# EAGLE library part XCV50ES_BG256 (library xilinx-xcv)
xcv50es_bg256 edit this description Auto generated by make-symbol-device-package-bsdl.ulp Rev. 26 Source: xcv50es_bg256.bsd
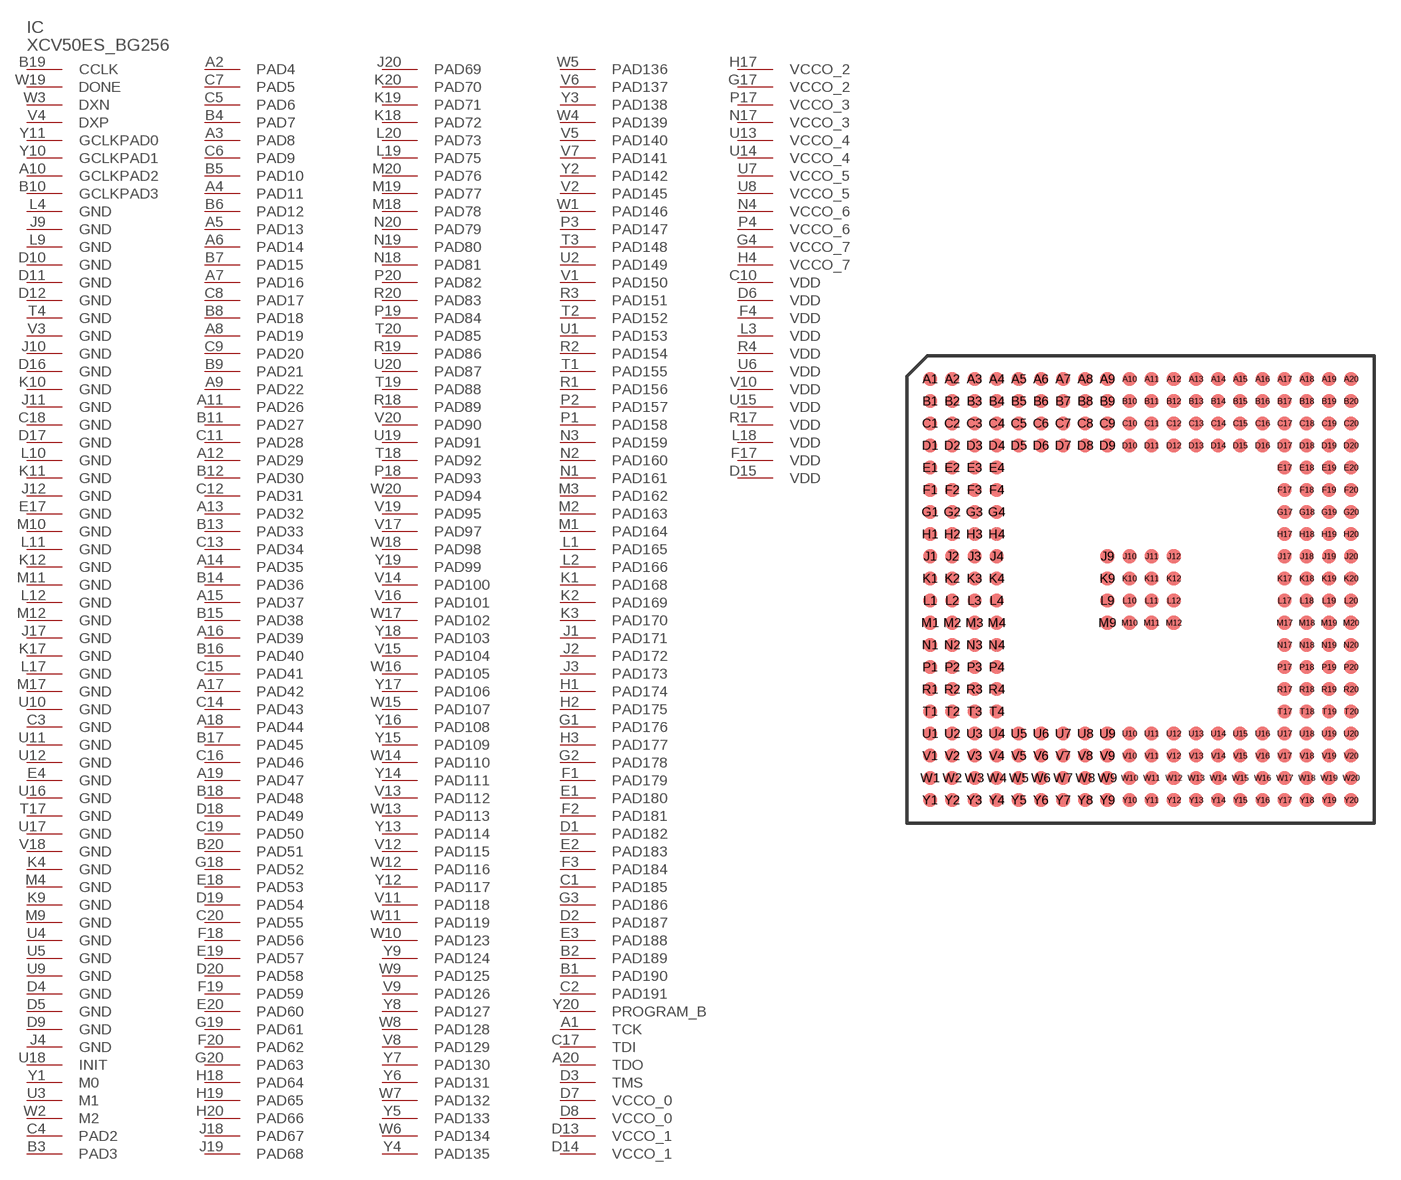
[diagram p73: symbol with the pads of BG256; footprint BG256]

Designator prefix IC

## XCV50ES_BG256 (OC_FARNELL: unknown; OC_NEWARK: unknown)  [BG256]
A1  TCK  in
A2  PAD4
A3  PAD8
A4  PAD11
A5  PAD13
A6  PAD14
A7  PAD16
A8  PAD19
A9  PAD22
A10  GCLKPAD2  in
A11  PAD26
A12  PAD29
A13  PAD32
A14  PAD35
A15  PAD37
A16  PAD39
A17  PAD42
A18  PAD44
A19  PAD47
A20  TDO  out
B1  PAD190
B2  PAD189
B3  PAD3
B4  PAD7
B5  PAD10
B6  PAD12
B7  PAD15
B8  PAD18
B9  PAD21
B10  GCLKPAD3  in
B11  PAD27
B12  PAD30
B13  PAD33
B14  PAD36
B15  PAD38
B16  PAD40
B17  PAD45
B18  PAD48
B19  CCLK
B20  PAD51
C1  PAD185
C2  PAD191
C3  GND  pwr
C4  PAD2
C5  PAD6
C6  PAD9
C7  PAD5
C8  PAD17
C9  PAD20
C10  VDD  pwr
C11  PAD28
C12  PAD31
C13  PAD34
C14  PAD43
C15  PAD41
C16  PAD46
C17  TDI  in
C18  GND  pwr
C19  PAD50
C20  PAD55
D1  PAD182
D2  PAD187
D3  TMS  in
D4  GND  pwr
D5  GND  pwr
D6  VDD  pwr
D7  VCCO_0  pwr
D8  VCCO_0  pwr
D9  GND  pwr
D10  GND  pwr
D11  GND  pwr
D12  GND  pwr
D13  VCCO_1  pwr
D14  VCCO_1  pwr
D15  VDD  pwr
D16  GND  pwr
D17  GND  pwr
D18  PAD49
D19  PAD54
D20  PAD58
E1  PAD180
E2  PAD183
E3  PAD188
E4  GND  pwr
E17  GND  pwr
E18  PAD53
E19  PAD57
E20  PAD60
F1  PAD179
F2  PAD181
F3  PAD184
F4  VDD  pwr
F17  VDD  pwr
F18  PAD56
F19  PAD59
F20  PAD62
G1  PAD176
G2  PAD178
G3  PAD186
G4  VCCO_7  pwr
G17  VCCO_2  pwr
G18  PAD52
G19  PAD61
G20  PAD63
H1  PAD174
H2  PAD175
H3  PAD177
H4  VCCO_7  pwr
H17  VCCO_2  pwr
H18  PAD64
H19  PAD65
H20  PAD66
J1  PAD171
J2  PAD172
J3  PAD173
J4  GND  pwr
J9  GND  pwr
J10  GND  pwr
J11  GND  pwr
J12  GND  pwr
J17  GND  pwr
J18  PAD67
J19  PAD68
J20  PAD69
K1  PAD168
K2  PAD169
K3  PAD170
K4  GND  pwr
K9  GND  pwr
K10  GND  pwr
K11  GND  pwr
K12  GND  pwr
K17  GND  pwr
K18  PAD72
K19  PAD71
K20  PAD70
L1  PAD165
L2  PAD166
L3  VDD  pwr
L4  GND  pwr
L9  GND  pwr
L10  GND  pwr
L11  GND  pwr
L12  GND  pwr
L17  GND  pwr
L18  VDD  pwr
L19  PAD75
L20  PAD73
M1  PAD164
M2  PAD163
M3  PAD162
M4  GND  pwr
M9  GND  pwr
M10  GND  pwr
M11  GND  pwr
M12  GND  pwr
M17  GND  pwr
M18  PAD78
M19  PAD77
M20  PAD76
N1  PAD161
N2  PAD160
N3  PAD159
N4  VCCO_6  pwr
N17  VCCO_3  pwr
N18  PAD81
N19  PAD80
N20  PAD79
P1  PAD158
P2  PAD157
P3  PAD147
P4  VCCO_6  pwr
P17  VCCO_3  pwr
P18  PAD93
P19  PAD84
P20  PAD82
R1  PAD156
R2  PAD154
R3  PAD151
R4  VDD  pwr
R17  VDD  pwr
R18  PAD89
R19  PAD86
R20  PAD83
T1  PAD155
T2  PAD152
T3  PAD148
T4  GND  pwr
T17  GND  pwr
T18  PAD92
T19  PAD88
T20  PAD85
U1  PAD153
U2  PAD149
U3  M1  in
U4  GND  pwr
U5  GND  pwr
U6  VDD  pwr
U7  VCCO_5  pwr
U8  VCCO_5  pwr
U9  GND  pwr
U10  GND  pwr
U11  GND  pwr
U12  GND  pwr
U13  VCCO_4  pwr
U14  VCCO_4  pwr
U15  VDD  pwr
U16  GND  pwr
U17  GND  pwr
U18  INIT
U19  PAD91
U20  PAD87
V1  PAD150
V2  PAD145
V3  GND  pwr
V4  DXP  pas
V5  PAD140
V6  PAD137
V7  PAD141
V8  PAD129
V9  PAD126
V10  VDD  pwr
V11  PAD118
V12  PAD115
V13  PAD112
V14  PAD100
V15  PAD104
V16  PAD101
V17  PAD97
V18  GND  pwr
V19  PAD95
V20  PAD90
W1  PAD146
W2  M2  in
W3  DXN  pas
W4  PAD139
W5  PAD136
W6  PAD134
W7  PAD132
W8  PAD128
W9  PAD125
W10  PAD123
W11  PAD119
W12  PAD116
W13  PAD113
W14  PAD110
W15  PAD107
W16  PAD105
W17  PAD102
W18  PAD98
W19  DONE
W20  PAD94
Y1  M0  in
Y2  PAD142
Y3  PAD138
Y4  PAD135
Y5  PAD133
Y6  PAD131
Y7  PAD130
Y8  PAD127
Y9  PAD124
Y10  GCLKPAD1  in
Y11  GCLKPAD0  in
Y12  PAD117
Y13  PAD114
Y14  PAD111
Y15  PAD109
Y16  PAD108
Y17  PAD106
Y18  PAD103
Y19  PAD99
Y20  PROGRAM_B  in

## Footprint BG256 (pad centres in mm)
xcv100_bg256_1532 edit this description Auto generated by make-symbol-device-package-bsdl.ulp Rev. 25 Source: xcv100_bg256_1532.bsd
smd 0.8 x 0.8: A1 -12.065,12.065; A2 -10.795,12.065; A3 -9.525,12.065; A4 -8.255,12.065; A5 -6.985,12.065; A6 -5.715,12.065; A7 -4.445,12.065; A8 -3.175,12.065; A9 -1.905,12.065; A10 -0.635,12.065; A11 0.635,12.065; A12 1.905,12.065; A13 3.175,12.065; A14 4.445,12.065; A15 5.715,12.065; A16 6.985,12.065; A17 8.255,12.065; A18 9.525,12.065; A19 10.795,12.065; A20 12.065,12.065; B1 -12.065,10.795; B2 -10.795,10.795; B3 -9.525,10.795; B4 -8.255,10.795; B5 -6.985,10.795; B6 -5.715,10.795; B7 -4.445,10.795; B8 -3.175,10.795; B9 -1.905,10.795; B10 -0.635,10.795; B11 0.635,10.795; B12 1.905,10.795; B13 3.175,10.795; B14 4.445,10.795; B15 5.715,10.795; B16 6.985,10.795; B17 8.255,10.795; B18 9.525,10.795; B19 10.795,10.795; B20 12.065,10.795; C1 -12.065,9.525; C2 -10.795,9.525; C3 -9.525,9.525; C4 -8.255,9.525; C5 -6.985,9.525; C6 -5.715,9.525; C7 -4.445,9.525; C8 -3.175,9.525; C9 -1.905,9.525; C10 -0.635,9.525; C11 0.635,9.525; C12 1.905,9.525; C13 3.175,9.525; C14 4.445,9.525; C15 5.715,9.525; C16 6.985,9.525; C17 8.255,9.525; C18 9.525,9.525; C19 10.795,9.525; C20 12.065,9.525; D1 -12.065,8.255; D2 -10.795,8.255; D3 -9.525,8.255; D4 -8.255,8.255; D5 -6.985,8.255; D6 -5.715,8.255; D7 -4.445,8.255; D8 -3.175,8.255; D9 -1.905,8.255; D10 -0.635,8.255; D11 0.635,8.255; D12 1.905,8.255; D13 3.175,8.255; D14 4.445,8.255; D15 5.715,8.255; D16 6.985,8.255; D17 8.255,8.255; D18 9.525,8.255; D19 10.795,8.255; D20 12.065,8.255; E1 -12.065,6.985; E2 -10.795,6.985; E3 -9.525,6.985; E4 -8.255,6.985; E17 8.255,6.985; E18 9.525,6.985; E19 10.795,6.985; E20 12.065,6.985; F1 -12.065,5.715; F2 -10.795,5.715; F3 -9.525,5.715; F4 -8.255,5.715; F17 8.255,5.715; F18 9.525,5.715; F19 10.795,5.715; F20 12.065,5.715; G1 -12.065,4.445; G2 -10.795,4.445; G3 -9.525,4.445; G4 -8.255,4.445; G17 8.255,4.445; G18 9.525,4.445; G19 10.795,4.445; G20 12.065,4.445; H1 -12.065,3.175; H2 -10.795,3.175; H3 -9.525,3.175; H4 -8.255,3.175; H17 8.255,3.175; H18 9.525,3.175; H19 10.795,3.175; H20 12.065,3.175; J1 -12.065,1.905; J2 -10.795,1.905; J3 -9.525,1.905; J4 -8.255,1.905; J9 -1.905,1.905; J10 -0.635,1.905; J11 0.635,1.905; J12 1.905,1.905; J17 8.255,1.905; J18 9.525,1.905; J19 10.795,1.905; J20 12.065,1.905; K1 -12.065,0.635; K2 -10.795,0.635; K3 -9.525,0.635; K4 -8.255,0.635; K9 -1.905,0.635; K10 -0.635,0.635; K11 0.635,0.635; K12 1.905,0.635; K17 8.255,0.635; K18 9.525,0.635; K19 10.795,0.635; K20 12.065,0.635; L1 -12.065,-0.635; L2 -10.795,-0.635; L3 -9.525,-0.635; L4 -8.255,-0.635; L9 -1.905,-0.635; L10 -0.635,-0.635; L11 0.635,-0.635; L12 1.905,-0.635; L17 8.255,-0.635; L18 9.525,-0.635; L19 10.795,-0.635; L20 12.065,-0.635; M1 -12.065,-1.905; M2 -10.795,-1.905; M3 -9.525,-1.905; M4 -8.255,-1.905; M9 -1.905,-1.905; M10 -0.635,-1.905; M11 0.635,-1.905; M12 1.905,-1.905; M17 8.255,-1.905; M18 9.525,-1.905; M19 10.795,-1.905; M20 12.065,-1.905; N1 -12.065,-3.175; N2 -10.795,-3.175; N3 -9.525,-3.175; N4 -8.255,-3.175; N17 8.255,-3.175; N18 9.525,-3.175; N19 10.795,-3.175; N20 12.065,-3.175; P1 -12.065,-4.445; P2 -10.795,-4.445; P3 -9.525,-4.445; P4 -8.255,-4.445; P17 8.255,-4.445; P18 9.525,-4.445; P19 10.795,-4.445; P20 12.065,-4.445; R1 -12.065,-5.715; R2 -10.795,-5.715; R3 -9.525,-5.715; R4 -8.255,-5.715; R17 8.255,-5.715; R18 9.525,-5.715; R19 10.795,-5.715; R20 12.065,-5.715; T1 -12.065,-6.985; T2 -10.795,-6.985; T3 -9.525,-6.985; T4 -8.255,-6.985; T17 8.255,-6.985; T18 9.525,-6.985; T19 10.795,-6.985; T20 12.065,-6.985; U1 -12.065,-8.255; U2 -10.795,-8.255; U3 -9.525,-8.255; U4 -8.255,-8.255; U5 -6.985,-8.255; U6 -5.715,-8.255; U7 -4.445,-8.255; U8 -3.175,-8.255; U9 -1.905,-8.255; U10 -0.635,-8.255; U11 0.635,-8.255; U12 1.905,-8.255; U13 3.175,-8.255; U14 4.445,-8.255; U15 5.715,-8.255; U16 6.985,-8.255; U17 8.255,-8.255; U18 9.525,-8.255; U19 10.795,-8.255; U20 12.065,-8.255; V1 -12.065,-9.525; V2 -10.795,-9.525; V3 -9.525,-9.525; V4 -8.255,-9.525; V5 -6.985,-9.525; V6 -5.715,-9.525; V7 -4.445,-9.525; V8 -3.175,-9.525; V9 -1.905,-9.525; V10 -0.635,-9.525; V11 0.635,-9.525; V12 1.905,-9.525; V13 3.175,-9.525; V14 4.445,-9.525; V15 5.715,-9.525; V16 6.985,-9.525; V17 8.255,-9.525; V18 9.525,-9.525; V19 10.795,-9.525; V20 12.065,-9.525; W1 -12.065,-10.795; W2 -10.795,-10.795; W3 -9.525,-10.795; W4 -8.255,-10.795; W5 -6.985,-10.795; W6 -5.715,-10.795; W7 -4.445,-10.795; W8 -3.175,-10.795; W9 -1.905,-10.795; W10 -0.635,-10.795; W11 0.635,-10.795; W12 1.905,-10.795; W13 3.175,-10.795; W14 4.445,-10.795; W15 5.715,-10.795; W16 6.985,-10.795; W17 8.255,-10.795; W18 9.525,-10.795; W19 10.795,-10.795; W20 12.065,-10.795; Y1 -12.065,-12.065; Y2 -10.795,-12.065; Y3 -9.525,-12.065; Y4 -8.255,-12.065; Y5 -6.985,-12.065; Y6 -5.715,-12.065; Y7 -4.445,-12.065; Y8 -3.175,-12.065; Y9 -1.905,-12.065; Y10 -0.635,-12.065; Y11 0.635,-12.065; Y12 1.905,-12.065; Y13 3.175,-12.065; Y14 4.445,-12.065; Y15 5.715,-12.065; Y16 6.985,-12.065; Y17 8.255,-12.065; Y18 9.525,-12.065; Y19 10.795,-12.065; Y20 12.065,-12.065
